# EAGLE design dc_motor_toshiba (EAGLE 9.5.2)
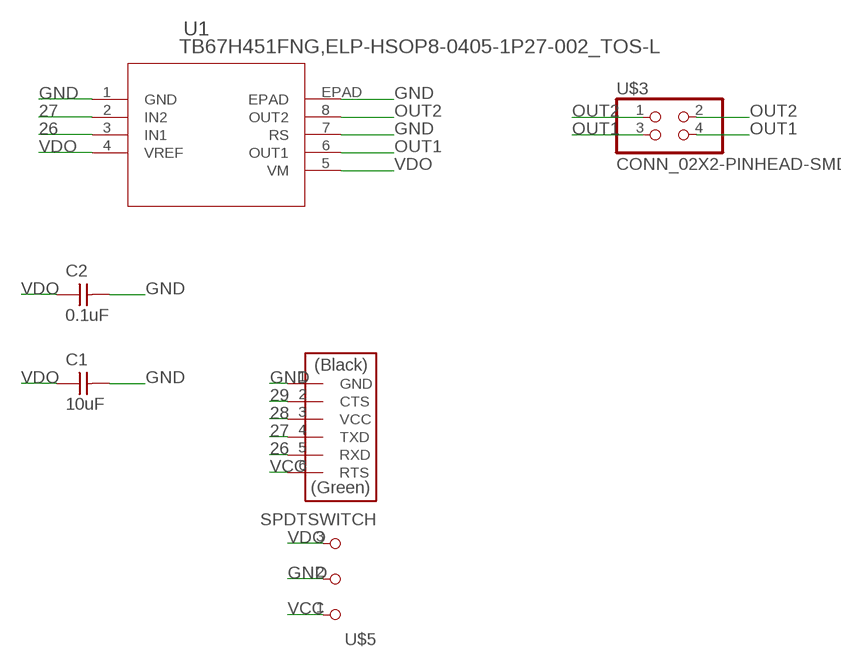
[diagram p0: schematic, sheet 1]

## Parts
C1  10uF  CAP_UNPOLARIZEDFAB  [C1206FAB]
C2  0.1uF  CAP_UNPOLARIZEDFAB  [C1206FAB]
U1  TB67H451FNG,ELP-HSOP8-0405-1P27-002_TOS-L  [P-HSOP8-0405-1P27-002_TOS-L-FAB]
U$1  CONN_06_FTDI-SMD-HEADER  [1X06SMD]
U$3  CONN_02X2-PINHEAD-SMD  [2X02SMD]
U$5  SPDTSWITCH  [SPDTSWITCH]

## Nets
26: U1.3(IN1) U$1.5(RXD)
27: U1.2(IN2) U$1.4(TXD)
28: U$1.3(VCC)
29: U$1.2(CTS)
GND: C1.2 C2.2 U1.1(GND) U1.7(RS) U1.EPAD U$1.1(GND) U$5.2
OUT1: U1.6(OUT1) U$3.3 U$3.4
OUT2: U1.8(OUT2) U$3.1 U$3.2
VCC: U$1.6(RTS) U$5.1
VDO: C1.1 C2.1 U1.4(VREF) U1.5(VM) U$5.3

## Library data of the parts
C1 C2 = fab:CAP_UNPOLARIZED
U1 = TB67H451FNG,EL_FAB:TB67H451FNG,EL; COPYRIGHT: Copyright (C) 2023 Ultra Librarian. All rights reserved.; MANUFACTURER_PART_NUMBER: TB67H451FNG,EL; MFR_NAME: Toshiba Electronic Devices & Storage Corp.
U$1 = fab:CONN_06_FTDI-SMD-HEADER
U$3 = fab:CONN_02X2-PINHEAD-SMD
U$5 = fab:SPDTSWITCH

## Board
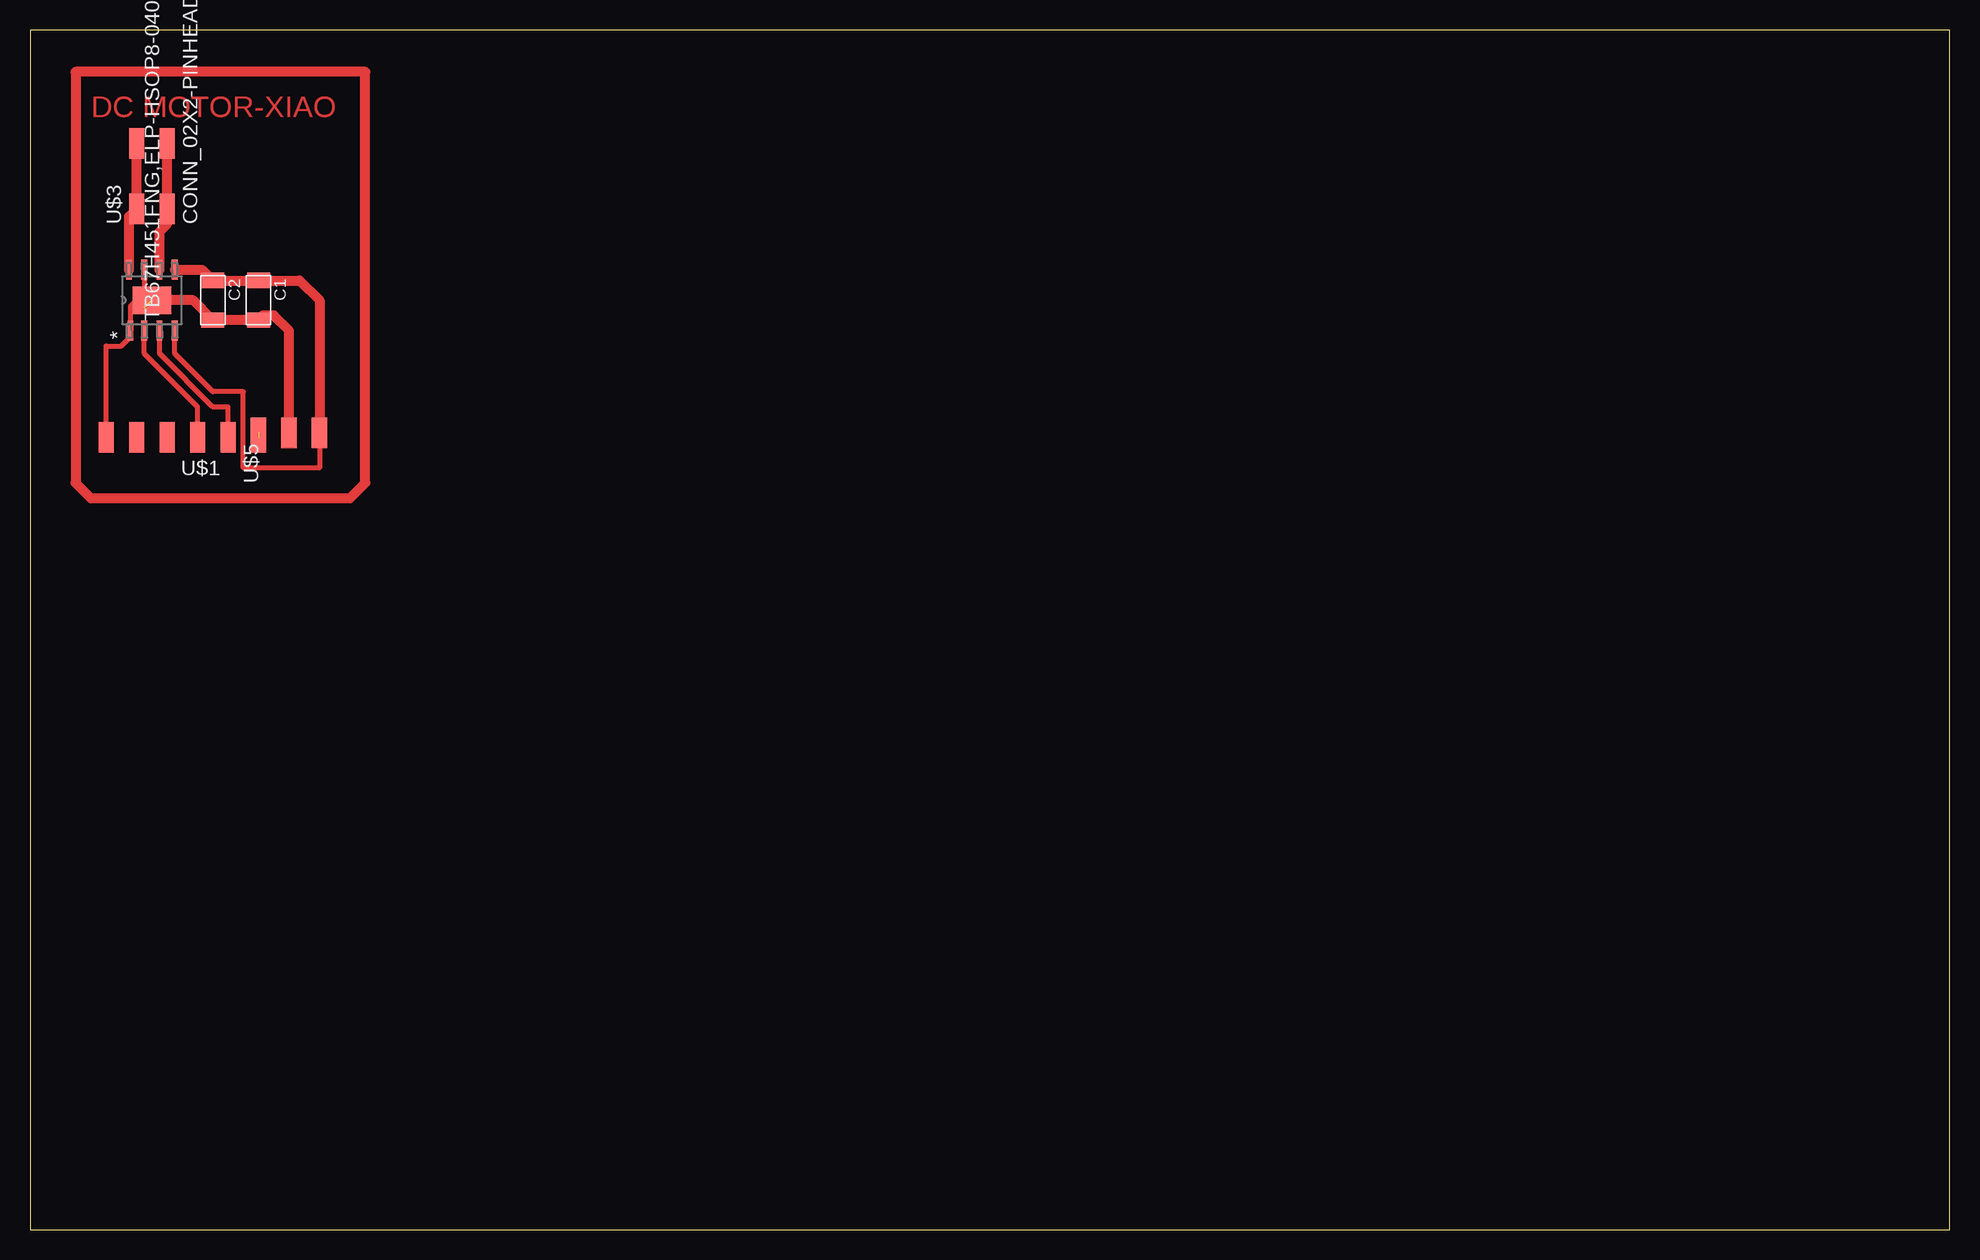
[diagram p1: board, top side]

Size 160 x 100 mm. Coordinates in mm from the lower left corner, seen from the top.
Outline: 0,0 160,0 160,100 0,100 0,0
Copper layers (1*16): Top 0.035mm / dielectric 1.5mm / Bottom 0.035mm
Design rules "default": minimum track width 6mil, minimum drill 0.35mm, track to track 6mil, track to pad 6mil, pad to pad 6mil, via to via 6mil, smd to smd 6mil, copper to edge 40mil, drill to drill 6mil, minimum pad ring 10mil, minimum via ring 8mil, stop-mask expansion 4mil, vias tented up to drill 0mil, thermal gap 10mil

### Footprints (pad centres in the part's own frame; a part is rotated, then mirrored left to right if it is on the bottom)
C1206FAB = smd 1.27 x 1.905: 1 -1.651,0; 2 1.651,0
P-HSOP8-0405-1P27-002_TOS-L-FAB = smd 1.676 x 0.483: 1 -2.54,1.778; 2 -2.54,0.635; 3 -2.54,-0.635; 4 -2.54,-1.905; 5 2.54,-1.905; 6 2.54,-0.635; 7 2.54,0.635; 8 2.54,1.905 | smd 2.286 x 3.2: EPAD 0,0
1X06SMD = smd 2.54 x 1.27: 1 0,6.35; 2 0,3.81; 3 0,1.27; 4 0,-1.27; 5 0,-3.81; 6 0,-6.35
2X02SMD = smd 2.54 x 1.27: 1 -2.54,1.27; 2 2.92,1.27; 3 -2.54,-1.27; 4 2.92,-1.27
SPDTSWITCH = smd 2.54 x 1.27: 1 0.38,2.54; 2 0.38,0; 3 0.38,-2.54

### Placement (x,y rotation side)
C1  19.05,77.47 270 top
C2  15.24,77.47 270 top
U1  10.16,77.47 90 top
U$1  12.7,66.04 90 top
U$3  10.16,87.63 90 top
U$5  21.59,66.04 90 top

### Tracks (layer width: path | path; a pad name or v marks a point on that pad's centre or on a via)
26
  Top 0.406: U$1.5 16.51,68.58 15.24,68.58 10.79,73.03 U1.3
27
  Top 0.406: U$1.4 13.97,68.58 9.53,73.03 U1.2
GND  (1 unrouted)
  Top 0.406: U$1.1 6.35,73.66 7.62,73.66 8.38,74.42 U1.1 8.38,76.96 8.89,77.47 | U1.7 9.53,78.11 8.89,77.47 | 8.89,77.47 9.53,76.83
  Top 0.813: U$5.2 21.59,74.93 20.32,76.2 19.43,76.2 C1.2 C2.2 13.59,77.47 U1.EPAD
N$1
  Top 0.813: 3.81,96.52 3.81,62.23 5.08,60.96 26.67,60.96 27.94,62.23 27.94,96.52 3.81,96.52
OUT1
  Top 0.813: U1.6 10.79,83.19 11.43,83.82 U$3.3 U$3.4
OUT2
  Top 0.813: U1.8 8.26,84.45 U$3.1 U$3.2
VCC  (1 unrouted)
VDO
  Top 0.406: U$5.3 24.13,63.5 17.78,63.5 17.78,69.85 15.24,69.85 12.06,73.03 U1.4
  Top 0.813: U1.5 14.35,80.01 C2.1 C1.1 22.48,79.12 24.13,77.47 U$5.3

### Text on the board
Top: DC MOTOR-XIAO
